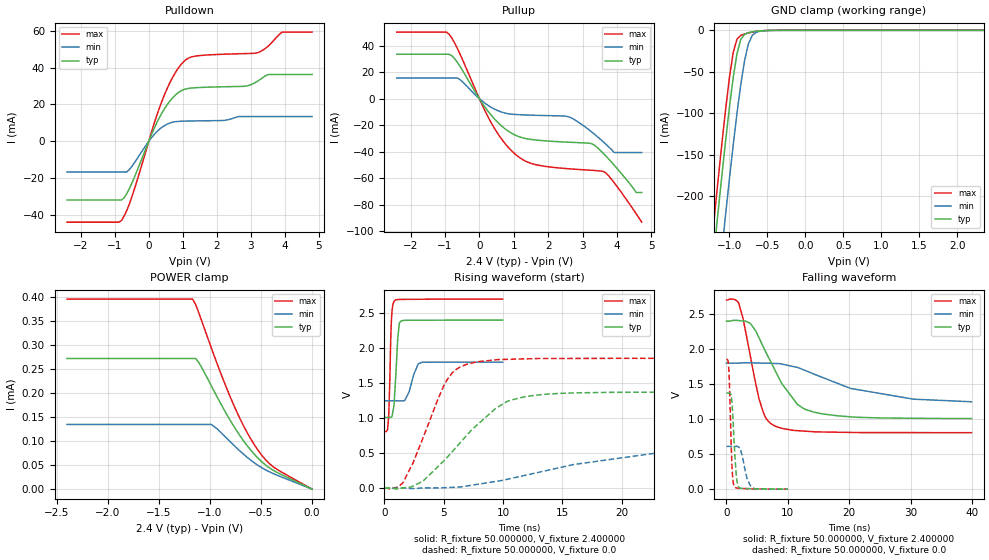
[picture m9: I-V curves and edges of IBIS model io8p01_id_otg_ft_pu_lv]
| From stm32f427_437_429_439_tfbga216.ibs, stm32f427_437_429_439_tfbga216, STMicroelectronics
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|   Model io8p01_id_otg_ft_pu_lv
[Model]  io8p01_id_otg_ft_pu_lv
Model_type I/O
Polarity   Non-Inverting
Enable   Active-Low
Vinl =   0.720000V
Vinh =   1.680000V
Vmeas =  1.200000V
Cref =   50.000000pF
Rref =   100.000000M
Vref =   0.0V
C_comp   2.229800pF   2.169700pF   2.325100pF
[Temperature Range]   25.000000   0.125000k   -40.000000
[Pullup Reference]   2.400000V   1.800000V   2.700000V
[Pulldown Reference]   0.0V   0.0V   0.0V
[POWER Clamp Reference]   2.400000V   1.800000V   2.700000V
[GND Clamp Reference]   0.0V   0.0V   0.0V
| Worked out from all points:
|   slope of the pulldown table from 0 to 0.36 V, typ, clamps not added: 25 ohm
|   slope of the pullup table from 0 to 0.36 V, typ, clamps not added: 27.7 ohm
|   GND clamp passes 1 mA (typ) near -0.62 V on its own axis
|   rising waveform, R_fixture 50.000000, V_fixture 2.400000: 20-80 % time 272ps typ, 607ps min, 181ps max; typ from 1.01 V to 2.4 V
|   rising waveform, R_fixture 50.000000, V_fixture 0.0: 20-80 % time 4.79ns typ, 12.2ns min, 2.63ns max; typ from 0.004 V to 1.37 V
|   falling waveform, R_fixture 50.000000, V_fixture 2.400000: 20-80 % time 5.37ns typ, 12.6ns min, 2.72ns max; typ from 2.4 V to 1.01 V
|   falling waveform, R_fixture 50.000000, V_fixture 0.0: 20-80 % time 527ps typ, 979ps min, 387ps max; typ from 1.37 V to 0.004 V
[Pulldown]
|Voltage   I(typ)   I(min)   I(max)
-2.4V     -31.73mA   -16.51mA   -43.74mA
-800mV    -31.73mA   -16.51mA   -42.87mA
-480mV    -21.97mA   -13.17mA   -29.21mA
80mV      3.63mA     1.966mA    5.014mA
480mV     18.15mA    8.737mA    26.02mA
800mV     25.37mA    10.72mA    37.77mA
1.12V     28.53mA    11.02mA    44.6mA
2.8V      29.84mA    13.46mA    47.53mA
3.2V      32.6mA     13.46mA    48.03mA
3.52V     36.23mA    13.46mA    51.75mA
3.92V     36.23mA    13.46mA    59.19mA
4.8V      36.23mA    13.46mA    59.19mA
[Pullup]
|Voltage   I(typ)   I(min)   I(max)
-2.4V     33.5mA     15.55mA    50.22mA
-960mV    33.5mA     15.55mA    50.22mA
-560mV    24.27mA    14.29mA    33.52mA
320mV     -11.75mA   -6.206mA   -17.08mA
960mV     -26.46mA   -11.81mA   -40.01mA
1.52V     -30.88mA   -12.51mA   -49.04mA
2.56V     -32.87mA   -13.48mA   -52.89mA
3.28V     -34.17mA   -25.52mA   -54.16mA
3.6V      -41.29mA   -32.61mA   -54.95mA
3.92V     -50.31mA   -40.7mA    -63.6mA
4.56V     -70.9mA    -40.7mA    -87.04mA
4.72V     -70.9mA    -40.7mA    -93.3mA
[GND_clamp]
|Voltage   I(typ)   I(min)   I(max)
-2.4V     -1.424A    -1.508A    -1.393A
-1.25V    -311.2mA   -401.9mA   -273.3mA
-1.2V     -265.4mA   -356.1mA   -227.2mA
-1.15V    -220.4mA   -310.8mA   -181.9mA
-1.1V     -176.3mA   -266.2mA   -137.9mA
-1.05V    -133.8mA   -222.5mA   -95.88mA
-950mV    -57.31mA   -138.9mA   -26.99mA
-900mV    -28.28mA   -100.4mA   -10.61mA
-850mV    -11.02mA   -65.55mA   -5.978mA
-750mV    -2.847mA   -16.51mA   -3.192mA
-600mV    -755.4uA   -1.17mA    -743.6uA
2.35V     0A         0A         0A
[POWER_clamp]
|Voltage   I(typ)   I(min)   I(max)
-2.4V     272.5uA    135uA      396.5uA
-1.17V    272.5uA    135uA      396.5uA
-1.14V    272.5uA    135uA      384.7uA
-1.11V    264.2uA    135uA      368uA
-990mV    216.8uA    135uA      296.5uA
-870mV    168.8uA    113.3uA    228.2uA
-750mV    125.6uA    88.19uA    167.1uA
-660mV    97.6uA     70.82uA    127.5uA
-570mV    73.91uA    55.62uA    94.12uA
-480mV    54.73uA    43.14uA    67.37uA
-390mV    40.65uA    33.48uA    48.23uA
0V        0A         0A         0A
[Ramp]
| variable   typ   min   max
dV/dt_r  0.82201/4.79105n   0.38518/13.04708n   1.10978/2.63063n
dV/dt_f  0.83370/5.37677n   0.32208/13.41905n   1.13507/2.71686n
R_load = 50.000000
[Rising Waveform]
R_fixture= 50.000000
V_fixture= 2.400000
V_fixture_min= 1.800000
V_fixture_max= 2.700000
|time   V(typ)   V(min)   V(max)
0s        1.011V     1.249V     809.2mV
260.3ps   1.011V     1.249V     835.8mV
340.3ps   1.011V     1.249V     994.1mV
600.6ps   1.02V      1.249V     2.446V
860.9ps   1.346V     1.249V     2.678V
1.121ns   2.146V     1.249V     2.693V
1.381ns   2.384V     1.247V     2.695V
1.722ns   2.396V     1.257V     2.695V
3.043ns   2.398V     1.789V     2.697V
9.97ns    2.4V       1.8V       2.7V
[Rising Waveform]
R_fixture= 50.000000
V_fixture= 0.0
V_fixture_min= 0.0
V_fixture_max= 0.0
|time   V(typ)   V(min)   V(max)
0s        3.754mV    3.294mV    4.214mV
1.602ns   9.053mV    3.122mV    93.83mV
3.283ns   108.3mV    6.701mV    735.6mV
5.125ns   412.2mV    10.64mV    1.503V
5.926ns   563.9mV    16.26mV    1.679V
6.967ns   761.1mV    34.31mV    1.77V
10.33ns   1.239V     128.3mV    1.84V
12.81ns   1.329V     221.9mV    1.851V
24.82ns   1.373V     548mV      1.854V
39.88ns   1.373V     613.5mV    1.854V
[Falling Waveform]
R_fixture= 50.000000
V_fixture= 2.400000
V_fixture_min= 1.800000
V_fixture_max= 2.700000
|time   V(typ)   V(min)   V(max)
0s        2.4V       1.8V       2.7V
2.002ns   2.407V     1.801V     2.653V
3.924ns   2.363V     1.805V     1.886V
5.285ns   2.165V     1.801V     1.299V
6.326ns   1.971V     1.8V       1.03V
7.608ns   1.749V     1.797V     917.5mV
11.53ns   1.213V     1.739V     837.5mV
14.09ns   1.105V     1.65V      822.4mV
20.26ns   1.035V     1.439V     812.2mV
39.88ns   1.011V     1.249V     809.2mV
[Falling Waveform]
R_fixture= 50.000000
V_fixture= 0.0
V_fixture_min= 0.0
V_fixture_max= 0.0
|time   V(typ)   V(min)   V(max)
0s        1.373V     613.5mV    1.854V
380.4ps   1.373V     613.6mV    1.722V
480.5ps   1.373V     613.6mV    1.525V
740.7ps   1.349V     613.5mV    737mV
981ps     1.132V     613.2mV    211.1mV
1.281ns   627.3mV    612.9mV    45.49mV
1.702ns   129.1mV    615mV      20.7mV
2.062ns   28.73mV    597.9mV    18mV
3.864ns   11.14mV    57.01mV    9.221mV
9.97ns    3.754mV    3.294mV    4.214mV
